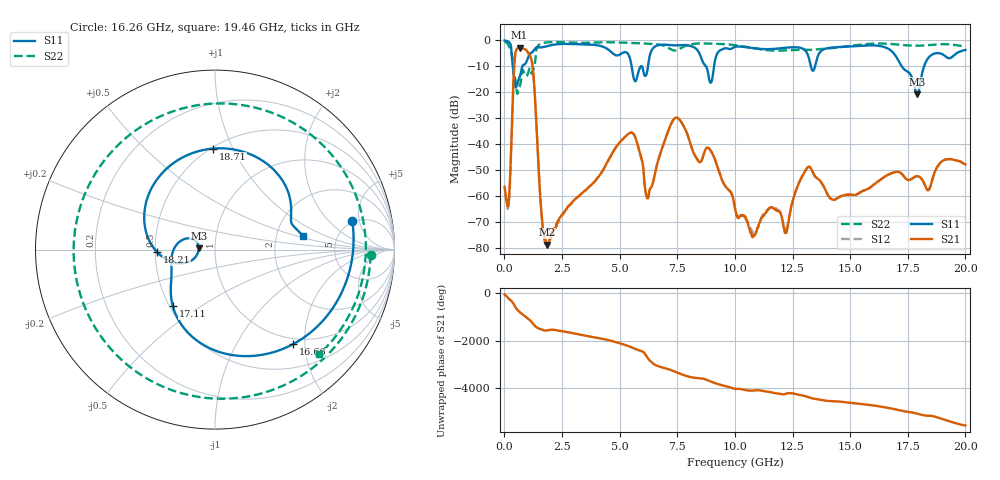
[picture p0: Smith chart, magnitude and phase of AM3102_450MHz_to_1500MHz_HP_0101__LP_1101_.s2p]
!Agilent Technologies,E8364B,MY43040894,A.07.50.67
!Agilent E8364B: A.07.50.67
!Date: Thursday, January 11, 2018 05:43:14
!Correction: S11(Full 2 Port(1,2))
!S21(Full 2 Port(1,2))
!S12(Full 2 Port(1,2))
!S22(Full 2 Port(1,2))
!S2P File: Measurements: S11, S21, S12, S22:
# Hz S  dB  R 50
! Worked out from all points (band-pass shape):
!   1601 points, 10 MHz to 20 GHz, reference 50 ohm
!   highest |S21| = -2.88 dB at 659.7 MHz (marker M1); lowest = -78.7 dB at 1.834 GHz (marker M2)
!   |S21| within 3 dB of the highest: 465.1 MHz to 1.101 GHz (635.9 MHz wide, 81.2 % of centre)
!   lowest |S11| = -20.8 dB at 17.9 GHz (marker M3), VSWR 1.20, Z = 41.7 + j0.571 ohm
!   |S11| at or under -10 dB: 365.9 MHz to 780.6 MHz (414.7 MHz wide, 72.3 % of centre); 5.52 GHz to 5.923 GHz (403 MHz wide, 7.04 % of centre); 17.24 GHz to 18.21 GHz (970.3 MHz wide, 5.48 % of centre)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
!   |S22| runs from -20.6 to -0.5 dB; largest |S21 - S12| = 0.0017
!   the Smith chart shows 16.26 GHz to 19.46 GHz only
!   S11 on the Smith chart (normalised r, x): 16.26 GHz: 4.77, +3.96; 16.66 GHz: 0.89, -1.76; 17.11 GHz: 0.52, -0.39; 18.21 GHz: 0.51, -0.02; 18.71 GHz: 0.51, +0.84; 19.46 GHz: 2.84, +0.57
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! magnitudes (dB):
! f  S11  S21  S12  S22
! 10 MHz  -0.1  -56.4  -58.6  -0.5
! 184.9 MHz  -0.6  -62.6  -63.7  -2.1
! 447.3 MHz  -15.8  -7.4  -7.4  -13.7
! 659.7 MHz  -14.2  -2.9  -2.9  -17.8
! 1.209 GHz  -4.6  -9.2  -9.2  -12.5
! 1.834 GHz  -2.3  -78.7  -79.0  -0.8
! 3.346 GHz  -1.5  -58.9  -59.1  -1.0
! 5.432 GHz  -6.5  -35.7  -35.7  -1.0
! 6.682 GHz  -1.9  -45.9  -45.9  -1.6
! 7.531 GHz  -1.9  -30.0  -30.0  -3.6
! 10.01 GHz  -2.5  -64.6  -64.5  -1.9
! 12.22 GHz  -2.8  -73.9  -72.7  -3.9
! 13.34 GHz  -11.3  -50.0  -50.0  -3.7
! 16.26 GHz  -2.1  -54.0  -54.0  -1.2
! 16.66 GHz  -3.3  -51.6  -51.6  -1.3
! 16.68 GHz  -3.4  -51.6  -51.6  -1.3
! 17.11 GHz  -8.1  -50.7  -50.7  -1.7
! 17.9 GHz  -20.8  -52.2  -52.3  -2.1
! 18.21 GHz  -9.8  -55.0  -55.2  -2.0
! 18.71 GHz  -5.0  -49.8  -49.8  -1.6
! 19.46 GHz  -6.1  -45.9  -45.9  -1.7
! 20 GHz  -3.7  -47.7  -47.7  -2.4
